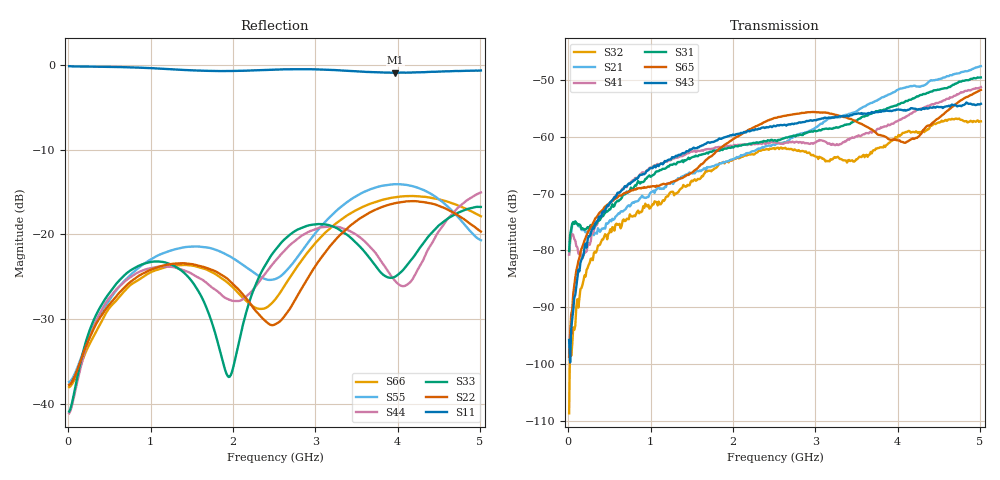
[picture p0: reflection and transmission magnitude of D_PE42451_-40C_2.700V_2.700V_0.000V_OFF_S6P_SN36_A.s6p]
! Device ID: PE42451
! Serial: 36
! Insertion: A
! Temp: -40C
! VDD: 2.700
! Control_Hi: 100.000
! Control_Lo: 0.000
! Logic State: OFF
! Port 1: RFC
! Port 2: RF1
! Port 3: RF2
! Port 4: RF3
! Port 5: RF4
! Port 6: RF5
! V1 = 0.00
! V2 = 2.70
! V3 = 2.70
! V4 = 0.00
! IDD: 1.073120e-05
#  Hz  S  RI  R  50
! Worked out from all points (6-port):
!   401 points, 10 MHz to 5.01 GHz, reference 50 ohm
!   strongest paths, dB at 10 MHz, 1.26 GHz, 2.51 GHz, 3.76 GHz, 5.01 GHz:
!     S43: -95.8, -63.6, -58.1, -55.6, -54.2
!     S65: -98.8, -67.9, -56.7, -59.6, -51.7
!     S31: -80.1, -64.9, -60.6, -55.5, -49.5
!     S41: -80.7, -63.9, -61.0, -58.6, -51.2
!     S21: -80.7, -68.0, -61.4, -53.5, -47.5
!     S32: -108.7, -69.7, -62.2, -62.0, -57.3
!   lowest |S11| = -0.9 dB at 3.973 GHz (marker M1), VSWR 19.60, Z = 2.78 - j14.9 ohm
!   |S11| at or under -10 dB: nowhere
